FUNCTION_BLOCK FB_DO_IED_LD1_ATCC1_LocKey EXTENDS FB_AcsiCommonDataClass
VAR_INPUT
	stVal: FB_AcsiBATypeBOOLEAN := (fc:=ACSI_FC_ST, TrgOp:=ACSI_TrgOp_dchg, bLinkResult:=THIS^.AddDataToContainer(ipData:=stVal));
	q: FB_AcsiDATypeQuality := (fc:=ACSI_FC_ST, TrgOp:=ACSI_TrgOp_qchg, bLinkResult:=THIS^.AddDataToContainer(ipData:=q));
	t: FB_AcsiDATypeTimeStamp := (fc:=ACSI_FC_ST, bLinkResult:=THIS^.AddDataToContainer(ipData:=t));
END_VAR
VAR
END_VAR

END_FUNCTION_BLOCK
